﻿FUNCTION "Called_Function" : Void
VERSION : 0.1
   VAR_INPUT
      Input : Bool;
   END_VAR

BEGIN
NETWORK
TITLE =

END_FUNCTION


FUNCTION_BLOCK "Function_Call2"
VERSION : 0.1
   VAR_INPUT
      In1 : Bool;
   END_VAR

BEGIN
NETWORK
TITLE =
      CALL "__CPROVER_assert"
      (  condition             := TRUE
      );

      CALL "__CPROVER_assume"
      (  condition             := #In1
      );

      CALL "__CPROVER_assert"
      (  condition             := #In1
      );

      CALL "Called_Function"
      (  Input                 := #In1
      );

END_FUNCTION_BLOCK

